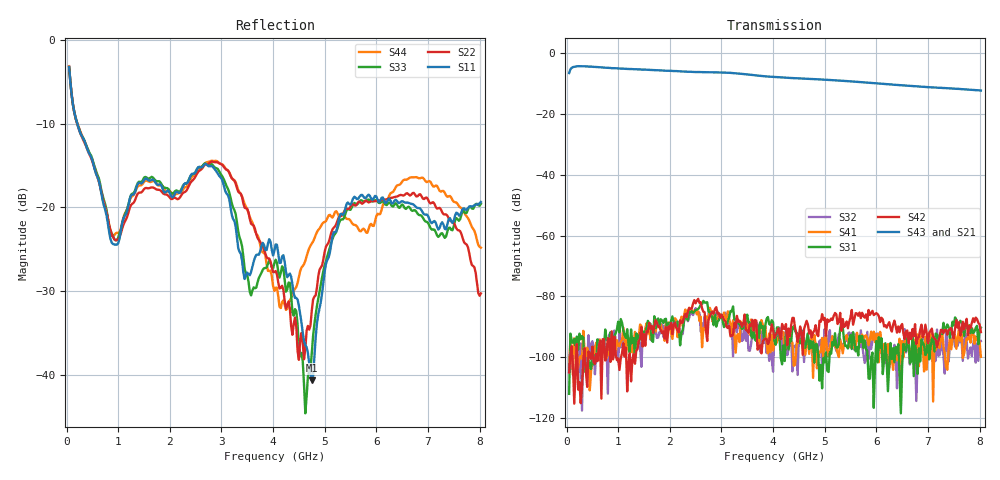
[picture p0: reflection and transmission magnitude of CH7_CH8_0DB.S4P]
!Agilent Technologies,E5071C,MY46316741,A.11.02
!Date: Mon Jun 01 10:31:12 2026
!Data & Calibration Information:
!1:CH7 INPUT 2:CH7 OUTPUT 3:CH8 INPUT 4:CH8 OUTPUT
!Freq	S11:SOLT4(ON)	S12:SOLT4(ON)	S13:SOLT4(ON)	S14:SOLT4(ON)
!	S21:SOLT4(ON)	S22:SOLT4(ON)	S23:SOLT4(ON)	S24:SOLT4(ON)
!	S31:SOLT4(ON)	S32:SOLT4(ON)	S33:SOLT4(ON)	S34:SOLT4(ON)
!	S41:SOLT4(ON)	S42:SOLT4(ON)	S43:SOLT4(ON)	S44:SOLT4(ON)
!PortZ  Port1:50+j0  Port2:50+j0  Port3:50+j0  Port4:50+j0
!Above PortZ is port z conversion or system Z0 setting when saving the data.
!When reading, reference impedance value at option line is always used.
# Hz S dB R 50
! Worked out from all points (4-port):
!   320 points, 50 MHz to 8.025 GHz, reference 50 ohm
!   strongest paths, dB at 50 MHz, 2.05 GHz, 4.05 GHz, 6.05 GHz, 8.025 GHz:
!     S43: -6.4, -5.7, -7.8, -9.9, -12.2
!     S21: -6.5, -5.8, -7.9, -10.1, -12.4
!     S42: -105.0, -92.4, -92.7, -86.5, -91.7
!     S31: -112.0, -86.5, -95.9, -93.4, -90.2
!     S41: -103.3, -94.0, -92.8, -101.6, -99.9
!     S32: -104.9, -88.9, -92.7, -92.2, -94.7
!   lowest |S11| = -40.7 dB at 4.75 GHz (marker M1), VSWR 1.02, Z = 50.3 + j0.876 ohm
!   |S11| at or under -10 dB: 209.2 MHz to end of sweep
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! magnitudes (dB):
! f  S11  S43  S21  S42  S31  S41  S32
! 50 MHz  -3.2  -6.4  -6.5  -105.0  -112.0  -103.3  -104.9
! 875 MHz  -24.2  -4.8  -4.8  -91.5  -93.5  -95.1  -98.9
! 2.825 GHz  -15.1  -6.2  -6.2  -85.0  -87.0  -88.2  -85.0
! 4.15 GHz  -26.6  -7.9  -8.1  -94.1  -100.3  -92.4  -94.0
! 4.75 GHz  -40.7  -8.4  -8.5  -93.5  -96.9  -91.8  -92.4
! 5.425 GHz  -19.6  -9.1  -9.2  -88.2  -96.2  -92.7  -94.4
! 8.025 GHz  -19.3  -12.2  -12.4  -91.7  -90.2  -99.9  -94.7
